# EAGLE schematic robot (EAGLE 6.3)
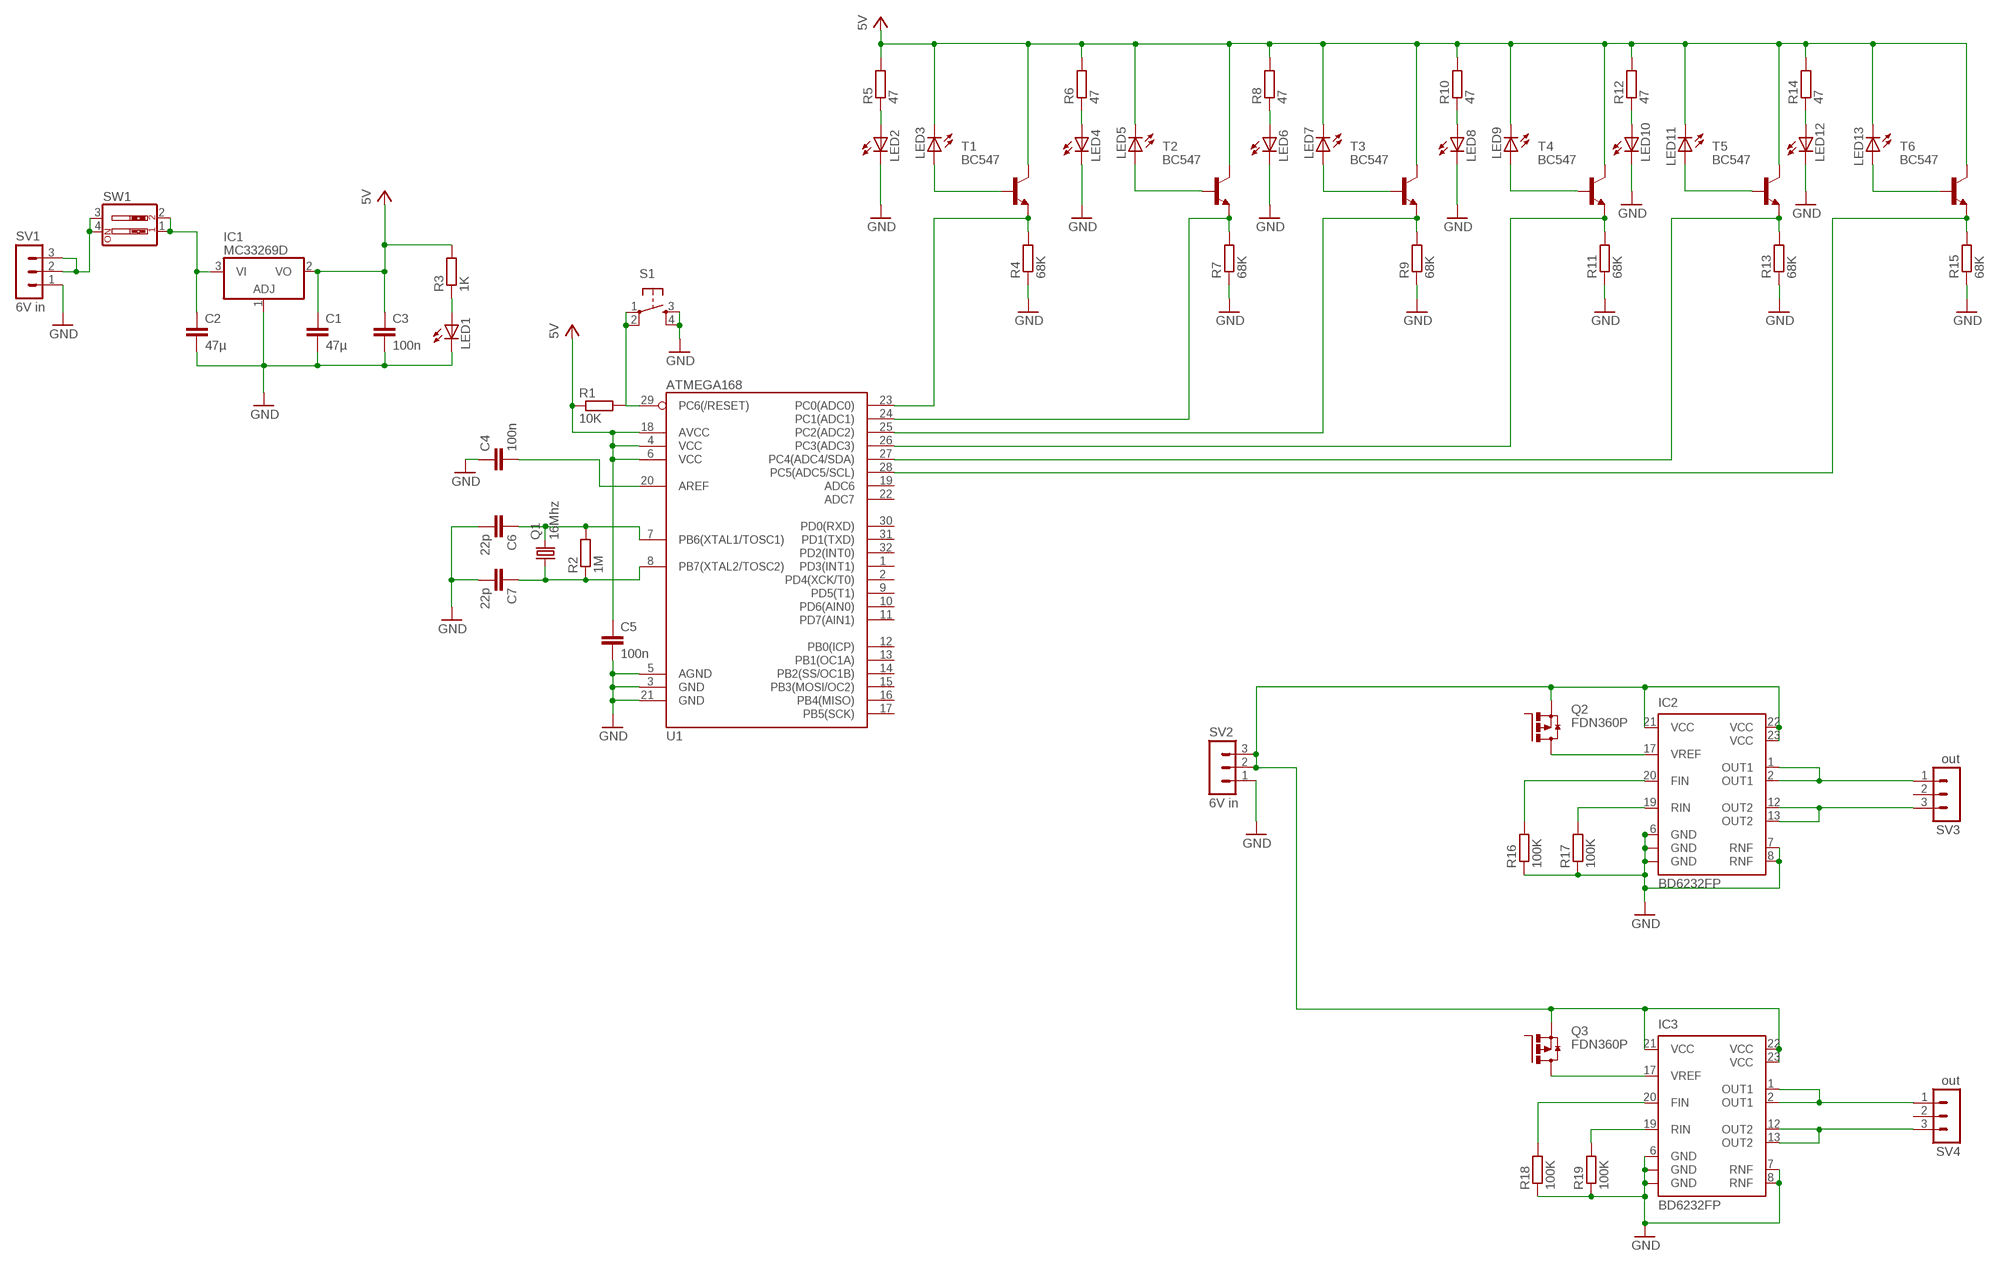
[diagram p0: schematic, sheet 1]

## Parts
C1  47µ  C2.5/5  [C2.5-5]
C2  47µ  C2.5/5  [C2.5-5]
C3  100n  C-EUC0805K  [C0805K]
C4  100n  C-EUC0805K  [C0805K]
C5  100n  C-EUC0805K  [C0805K]
C6  22p  C2.5/5  [C2.5-5]
C7  22p  C2.5/5  [C2.5-5]
IC1  MC33269D  [DPACK]
IC2  BD6232FP  [HSOP25]
IC3  BD6232FP  [HSOP25]
LED1  LEDCHIP-LED0805  [CHIP-LED0805]
LED2  LED5MM  [LED5MM]
LED3  LED5MM  [LED5MM]
LED4  LED5MM  [LED5MM]
LED5  LED5MM  [LED5MM]
LED6  LED5MM  [LED5MM]
LED7  LED5MM  [LED5MM]
LED8  LED5MM  [LED5MM]
LED9  LED5MM  [LED5MM]
LED10  LED5MM  [LED5MM]
LED11  LED5MM  [LED5MM]
LED12  LED5MM  [LED5MM]
LED13  LED5MM  [LED5MM]
Q1  16Mhz  CRYSTALHC49U-V  [HC49U-V]
Q2  FDN360P  [SUPER-SOT3]
Q3  FDN360P  [SUPER-SOT3]
R1  10K  R-EU_M1206  [M1206]
R2  1M  R-EU_M1206  [M1206]
R3  1K  R-EU_M1206  [M1206]
R4  68K  R-EU_M1206  [M1206]
R5  47  R-EU_M1206  [M1206]
R6  47  R-EU_M1206  [M1206]
R7  68K  R-EU_M1206  [M1206]
R8  47  R-EU_M1206  [M1206]
R9  68K  R-EU_M1206  [M1206]
R10  47  R-EU_M1206  [M1206]
R11  68K  R-EU_M1206  [M1206]
R12  47  R-EU_M1206  [M1206]
R13  68K  R-EU_M1206  [M1206]
R14  47  R-EU_M1206  [M1206]
R15  68K  R-EU_M1206  [M1206]
R16  100K  R-EU_M1206  [M1206]
R17  100K  R-EU_M1206  [M1206]
R18  100K  R-EU_M1206  [M1206]
R19  100K  R-EU_M1206  [M1206]
S1  TAC_SWITCHSMD  [TACTILE_SWITCH_SMD]
SV1  6V in  MA03-1  [MA03-1]
SV2  6V in  MA03-1  [MA03-1]
SV3  out  MA03-1  [MA03-1]
SV4  out  MA03-1  [MA03-1]
SW1  SW_DIP-2  [EDG-02]
T1  BC547  [TO92]
T2  BC547  [TO92]
T3  BC547  [TO92]
T4  BC547  [TO92]
T5  BC547  [TO92]
T6  BC547  [TO92]
U1  ATMEGA168  [TQFP32-08]

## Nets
GND: C1.2 C2.2 C3.2 C4.1 C5.2 C6.2 C7.2 IC1.1(ADJ) IC2.6(GND) IC2.7(RNF) IC2.8(RNF) IC2.GND@1(GND) IC2.GND@2(GND) IC3.6(GND) IC3.7(RNF) IC3.8(RNF) IC3.GND@1(GND) IC3.GND@2(GND) LED1.C LED2.K(C) LED4.K(C) LED6.K(C) LED8.K(C) LED10.K(C) LED12.K(C) R4.1 R7.1 R9.1 R11.1 R13.1 R15.1 R16.1 R17.1 R18.1 R19.1 S1.3 S1.4 SV1.1 SV2.1 U1.3(GND) U1.5(AGND) U1.21(GND)
N$1: C2.1 IC1.3(VI) SW1.1 SW1.2
N$2: R1.2 S1.1 S1.2 U1.29(PC6(/RESET))
N$3: C4.2 U1.20(AREF)
N$4: C6.1 Q1.2 R2.2 U1.7(PB6(XTAL1/TOSC1))
N$5: C7.1 Q1.1 R2.1 U1.8(PB7(XTAL2/TOSC2))
N$6: LED1.A R3.1
N$7: R4.2 T1.1(E) U1.23(PC0(ADC0))
N$8: SV1.2 SV1.3 SW1.3 SW1.4
N$9: R9.2 T3.1(E) U1.25(PC2(ADC2))
N$10: LED2.A R5.1
N$11: LED3.A T1.2(B)
N$12: R7.2 T2.1(E) U1.24(PC1(ADC1))
N$13: R11.2 T4.1(E) U1.26(PC3(ADC3))
N$14: LED5.A T2.2(B)
N$15: LED4.A R6.1
N$16: LED8.A R10.1
N$17: LED6.A R8.1
N$18: LED7.A T3.2(B)
N$19: LED9.A T4.2(B)
N$20: IC3.1(OUT1) IC3.2(OUT1) SV4.1
N$21: IC3.12(OUT2) IC3.13(OUT2) SV4.3
N$22: IC2.1(OUT1) IC2.2(OUT1) SV3.1
N$23: IC2.12(OUT2) IC2.13(OUT2) SV3.3
N$24: IC2.19(RIN) R17.2
N$25: IC2.20(FIN) R16.2
N$26: IC3.19(RIN) R19.2
N$27: R13.2 T5.1(E) U1.27(PC4(ADC4/SDA))
N$28: LED11.A T5.2(B)
N$29: LED10.A R12.1
N$30: IC3.20(FIN) R18.2
N$31: IC2.17(VREF) Q2.3(D)
N$32: LED12.A R14.1
N$33: LED13.A T6.2(B)
N$34: R15.2 T6.1(E) U1.28(PC5(ADC5/SCL))
N$35: IC2.21(VCC) IC2.22(VCC) IC2.23(VCC) IC3.21(VCC) IC3.22(VCC) IC3.23(VCC) Q2.2(S) Q3.2(S) SV2.2 SV2.3
N$38: IC3.17(VREF) Q3.3(D)
VCC: C1.1 C3.1 C5.1 IC1.2(VO) LED3.K(C) LED5.K(C) LED7.K(C) LED9.K(C) LED11.K(C) LED13.K(C) R1.1 R3.2 R5.2 R6.2 R8.2 R10.2 R12.2 R14.2 T1.3(C) T2.3(C) T3.3(C) T4.3(C) T5.3(C) T6.3(C) U1.4(VCC) U1.6(VCC) U1.18(AVCC) ; supply symbol labelled 5V
Unconnected: Q2.1(G) Q3.1(G) SV3.2 SV4.2 U1.1(PD3(INT1)) U1.2(PD4(XCK/T0)) U1.9(PD5(T1)) U1.10(PD6(AIN0)) U1.11(PD7(AIN1)) U1.12(PB0(ICP)) U1.13(PB1(OC1A)) U1.14(PB2(SS/OC1B)) U1.15(PB3(MOSI/OC2)) U1.16(PB4(MISO)) U1.17(PB5(SCK)) U1.19(ADC6) U1.22(ADC7) U1.30(PD0(RXD)) U1.31(PD1(TXD)) U1.32(PD2(INT0))

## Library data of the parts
C1 C2 C6 C7 = capacitor-wima:C: CAPACITOR
C3-C5 = rcl:C-EU: CAPACITOR, European symbol
IC1 = linear:MC33269?*: Adjustable Output Low Dropout Voltage Regulator 800 mA Source: http://www.onsemi.com/pub/Collateral/MC33269-D.PDF
IC2 IC3 = rohm:BD6232FP: H-bridge driver for brush motors Source: http://www.rohm.com/products/databook/motor/pdf/bd623x_series-e.pdf; MPN: BD6232FP-E2; OC_FARNELL: 1716266; OC_NEWARK: 15R0531
LED1-LED13 = led:LED: LED
Q1 = crystal:CRYSTAL: CRYSTAL; OC_FARNELL: 1666969; OC_NEWARK: unknown
Q2 Q3 = transistor-power:FDN360P: Single P-Channel, PowerTrench (R) MOSFET Source: http://www.fairchildsemi.com/ds/FD/FDN360P.pdf
R1-R19 = resistor:R-EU_: RESISTOR, European symbol
S1 = SparkFun:TAC_SWITCH: Momentary Switch Button commonly used for reset or general input. Spark Fun Electronics SKU : COM-00097
SV1-SV4 = con-lstb:MA03-1: PIN HEADER; OC_FARNELL: unknown; OC_NEWARK: unknown
SW1 = special:SW_DIP-2: DIP SWITCH
T1-T6 = transistor:BC547: NPN TRANSISTOR
U1 = SparkFun:ATMEGA168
